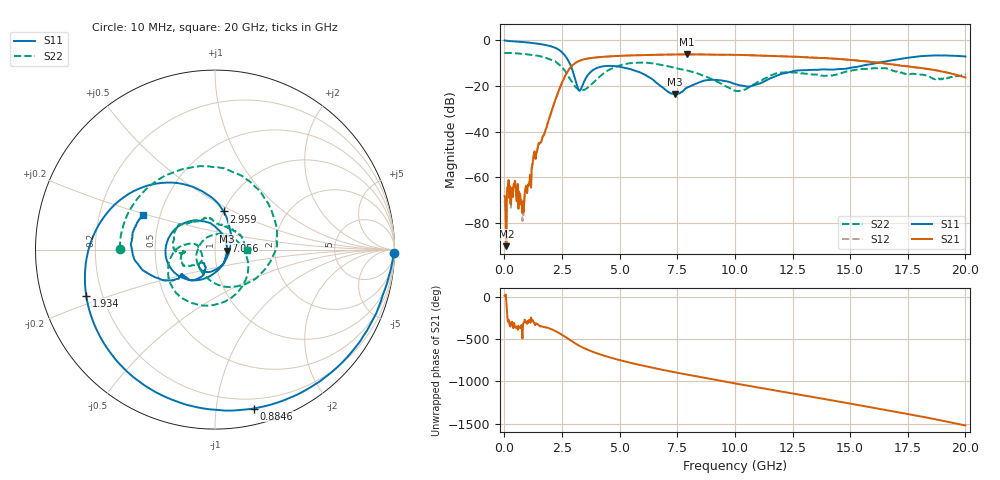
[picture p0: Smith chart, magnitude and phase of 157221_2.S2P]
!  2-Port S-parameters saved by WinCal
! VAR MeasName=S-Parameters (CALIBRATED_DATA) read from VNA (N5242A)
! VAR MeasDate=2015-5-26 16:47:21
! VAR NAME=157221_2
! VAR FILENAME=157221_2.S2P
! VAR DATE=2015-5-26 16:47:21
! VAR PHYS_PORTS=1,2
# Hz S DB R 50
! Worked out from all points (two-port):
!   801 points, 10 MHz to 20 GHz, reference 50 ohm
!   highest |S21| = -6.15 dB at 7.906 GHz (marker M1); lowest = -90.1 dB at 84.96 MHz (marker M2)
!   |S21| within 3 dB of the highest: 3.218 GHz to 15.61 GHz (12.39 GHz wide, 132 % of centre)
!   lowest |S11| = -23.4 dB at 7.406 GHz (marker M3), VSWR 1.14, Z = 57.2 - j0.887 ohm
!   |S11| at or under -10 dB: 2.829 GHz to 16.11 GHz (13.28 GHz wide, 140 % of centre)
!   |S22| runs from -22.3 to -5.5 dB; largest |S21 - S12| = 0.0092
!   S11 on the Smith chart (normalised r, x): 10 MHz: open; 884.6 MHz: 0.12, -1.27; 1.934 GHz: 0.14, -0.17; 2.959 GHz: 1.00, +0.45; 7.056 GHz: 1.12, +0.11; 20 GHz: 0.40, +0.19
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1e7  -0.04 -1.1  -68.13 12.9  -71.23 137.9  -5.53 179.5
8.49625e7  -0.17 -8.6  -90.09 -54.8  -88.90 167.4  -5.51 175.2
4.847625e8  -0.48 -43.0  -63.66 -5.1  -63.62 -7.4  -5.66 152.6
8.845625e8  -0.81 -76.3  -66.80 91.0  -66.76 83.3  -6.00 128.8
1.284362e9  -1.24 -108.1  -49.47 54.3  -49.34 54.6  -6.50 101.9
1.934038e9  -2.36 -160.3  -34.58 -12.8  -34.59 -13.2  -8.12 40.9
2.50875e9  -5.30 141.4  -18.33 -90.4  -18.34 -90.8  -11.84 -48.8
2.958525e9  -13.24 77.3  -10.86 -171.7  -10.86 -171.8  -18.53 -149.6
3.358325e9  -20.50 -61.8  -8.57 126.1  -8.56 125.9  -21.91 116.7
4.70765e9  -11.23 177.8  -6.93 -7.0  -6.93 -7.3  -12.08 -49.7
5.70715e9  -13.41 132.8  -6.53 -75.6  -6.54 -75.9  -9.81 -111.8
6.681662e9  -19.23 77.5  -6.28 -133.6  -6.28 -133.6  -10.50 -150.5
7.056475e9  -22.15 40.4  -6.23 -154.2  -6.23 -154.4  -11.21 -161.4
7.4063e9  -23.44 -6.6  -6.19 -173.2  -6.17 -173.5  -12.07 -170.4
7.90605e9  -20.80 -59.3  -6.15 160.4  -6.14 160.1  -13.13 -179.4
1.0005e10  -19.03 -138.5  -6.36 55.8  -6.36 55.3  -22.06 -172.2
1.145428e10  -16.99 -115.0  -6.79 -13.8  -6.76 -14.2  -15.75 -146.0
1.335332e10  -12.89 -137.9  -7.56 -103.5  -7.49 -103.8  -14.95 -177.4
1.485258e10  -12.35 -142.6  -8.44 -176.5  -8.41 -176.9  -13.64 -175.0
1.667666e10  -8.97 -153.5  -10.35 93.9  -10.32 93.5  -12.55 143.7
1.827586e10  -6.79 -175.7  -12.38 14.4  -12.36 13.1  -15.26 97.1
2e10  -7.07 154.1  -16.23 -81.8  -16.31 -83.5  -14.95 -0.3
